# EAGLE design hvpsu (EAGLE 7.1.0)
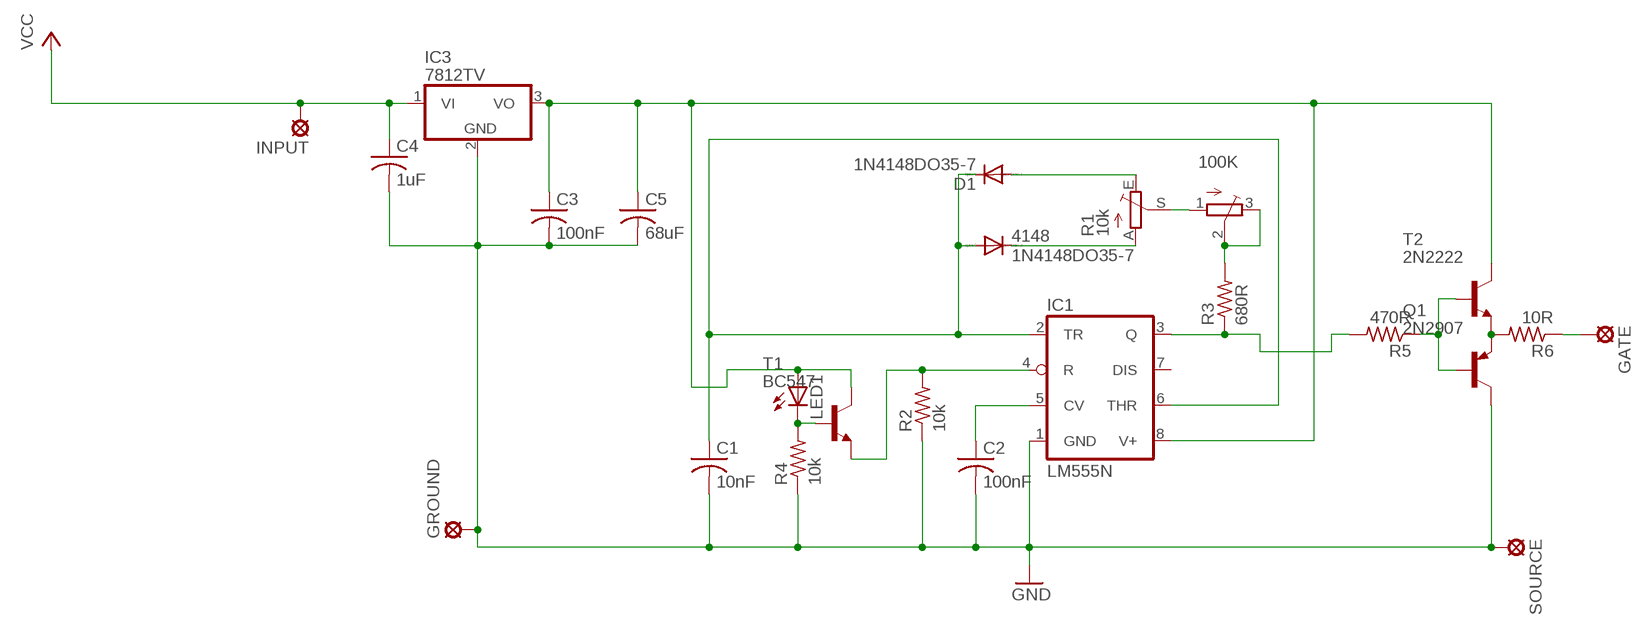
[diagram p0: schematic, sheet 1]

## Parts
100K  TRIMPOT3386  [TRIM-3386]
4148  1N4148DO35-7  [DO35-7]
C1  10nF  C-US050-024X044  [C050-024X044]
C2  100nF  C-US050-024X044  [C050-024X044]
C3  100nF  C-US025-025X050  [C025-025X050]
C4  1uF  C-US025-025X050  [C025-025X050]
C5  68uF  C-US025-025X050  [C025-025X050]
D1  1N4148DO35-7  [DO35-7]
GATE  LSP10  [LSP10]
GROUND  LSP10  [LSP10]
IC1  LM555N  [DIL08-ROUND]
IC3  7812TV  [TO220V]
INPUT  LSP10  [LSP10]
LED1  LED5MM  [LED5MM]
Q1  2N2907  [TO92-EBC-OVAL]
R1  10k  TRIM_EU-S64W  [S64W]
R2  10k  R-US_0204/7  [0204/7]
R3  680R  R-US_0204/7  [0204/7]
R4  10k  R-US_0204/7  [0204/7]
R5  470R  R-US_0204/7  [0204/7]
R6  10R  R-US_0204/7  [0204/7]
SOURCE  LSP10  [LSP10]
T1  BC547  [TO92]
T2  2N2222  [TO92-EBC-OVAL]

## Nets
4148: 4148.A C1.1 D1.C IC1.2(TR) IC1.6(THR)
GND: C1.2 C2.2 C3.2 C4.2 C5.2 GROUND.MP IC1.1(GND) IC3.2(GND) Q1.C R2.1 R4.1 SOURCE.MP
N$1: C2.1 IC1.5(CV)
N$2: IC1.3(Q) R3.1 R5.2
N$3: 100K.2(S) 100K.3(E) R3.2
N$4: 100K.1(A) R1.S
N$5: C3.1 C5.1 IC1.8(V+) IC3.3(VO) LED1.A T1.3(C) T2.C
N$6: 4148.C R1.A
N$7: D1.A R1.E
N$8: LED1.K(C) R4.2 T1.2(B)
N$9: IC1.4(R) R2.2 T1.1(E)
N$10: Q1.B R5.1 T2.B
N$11: Q1.E R6.2 T2.E
N$12: GATE.MP R6.1
VCC: C4.1 IC3.1(VI) INPUT.MP
Unconnected: IC1.7(DIS)

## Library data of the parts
100K = adafruit:TRIMPOT: SMT trimmer potentiometer part number TC33X http://www.ladyada.net/library/eagle
4148 D1 = diode:1N4148: DIODE
C1-C5 = adafruit:C-US: CAPACITOR, American symbol
GATE GROUND INPUT SOURCE = solpad:LSP10: SOLDER PAD
IC1 = adafruit:*555: TIMER Changed DIP package to have round (not oval) pin pads http://www.ladyada.net/library/pcb/eaglelibrary.html
IC3 = linear:78*: Positive VOLTAGE REGULATOR Source: http://cache.national.com/ds/LM/LM78L05.pdf http://www.fairchildsemi.com/ds/LM/LM7805.pdf
LED1 = adafruit:LED: LED
Q1 = adafruit:2N2907*: PNP Transistor Big Oval pads
R1 = pot:TRIM_EU-: POTENTIOMETER
R2-R6 = adafruit:R-US_: RESISTOR, American symbol
T1 = transistor:BC547: NPN TRANSISTOR
T2 = adafruit:2N2222: NPN TRANSISTOR Big oval pads

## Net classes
0 default: clearance 0.508 mm

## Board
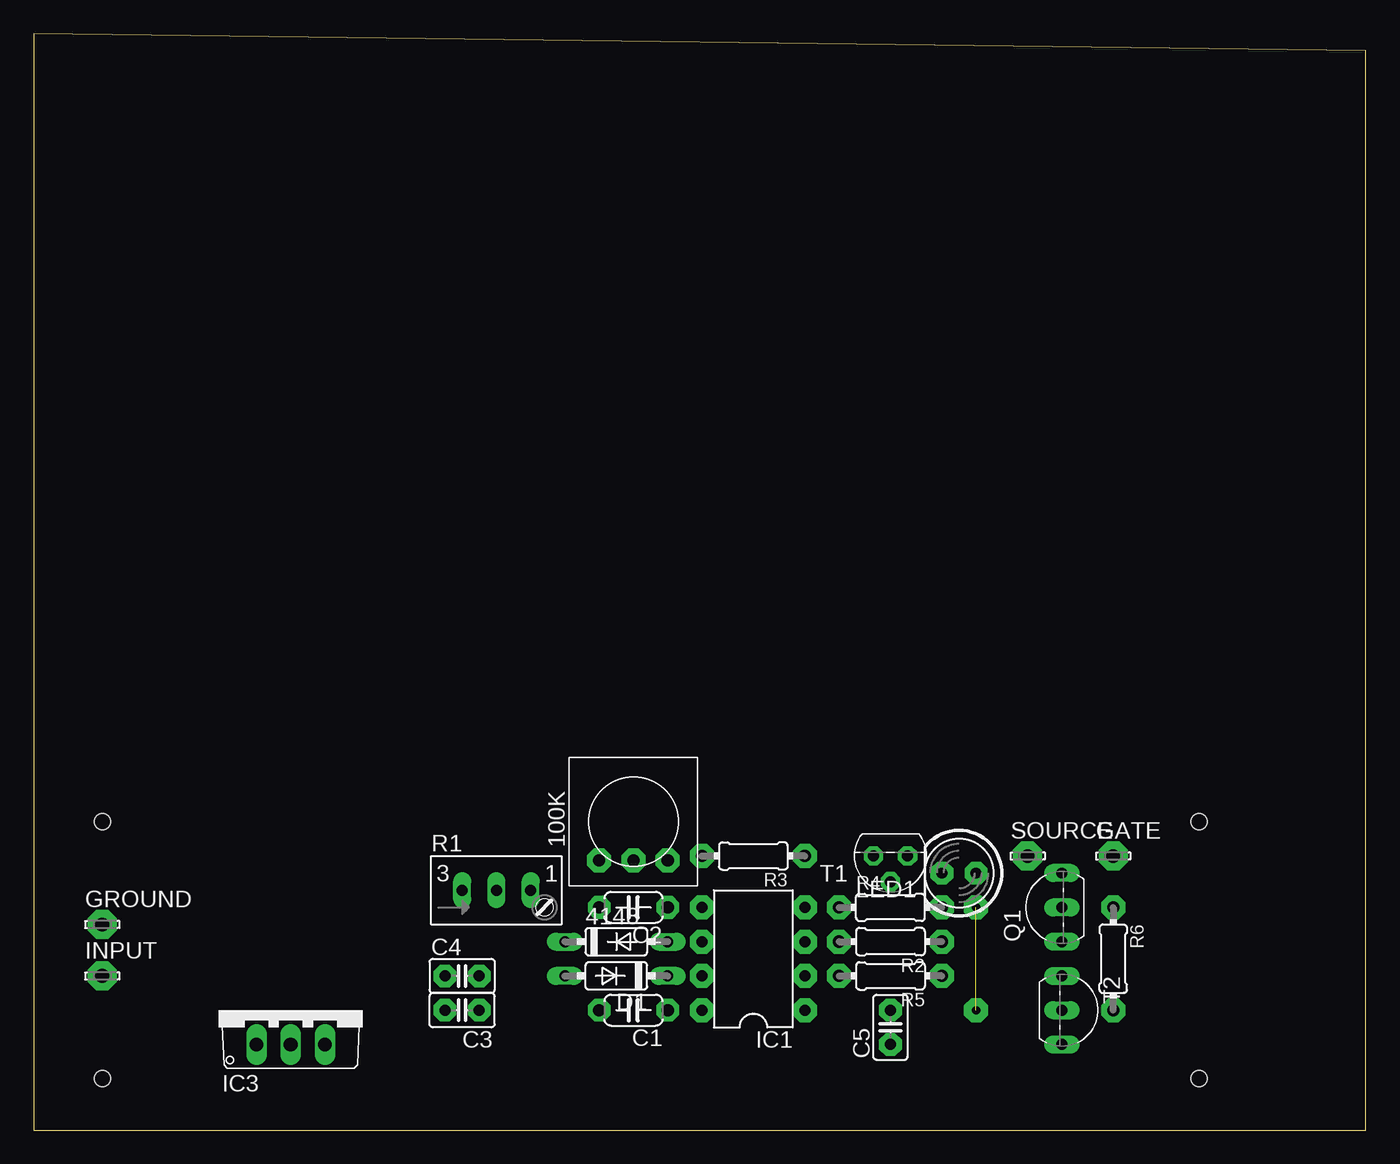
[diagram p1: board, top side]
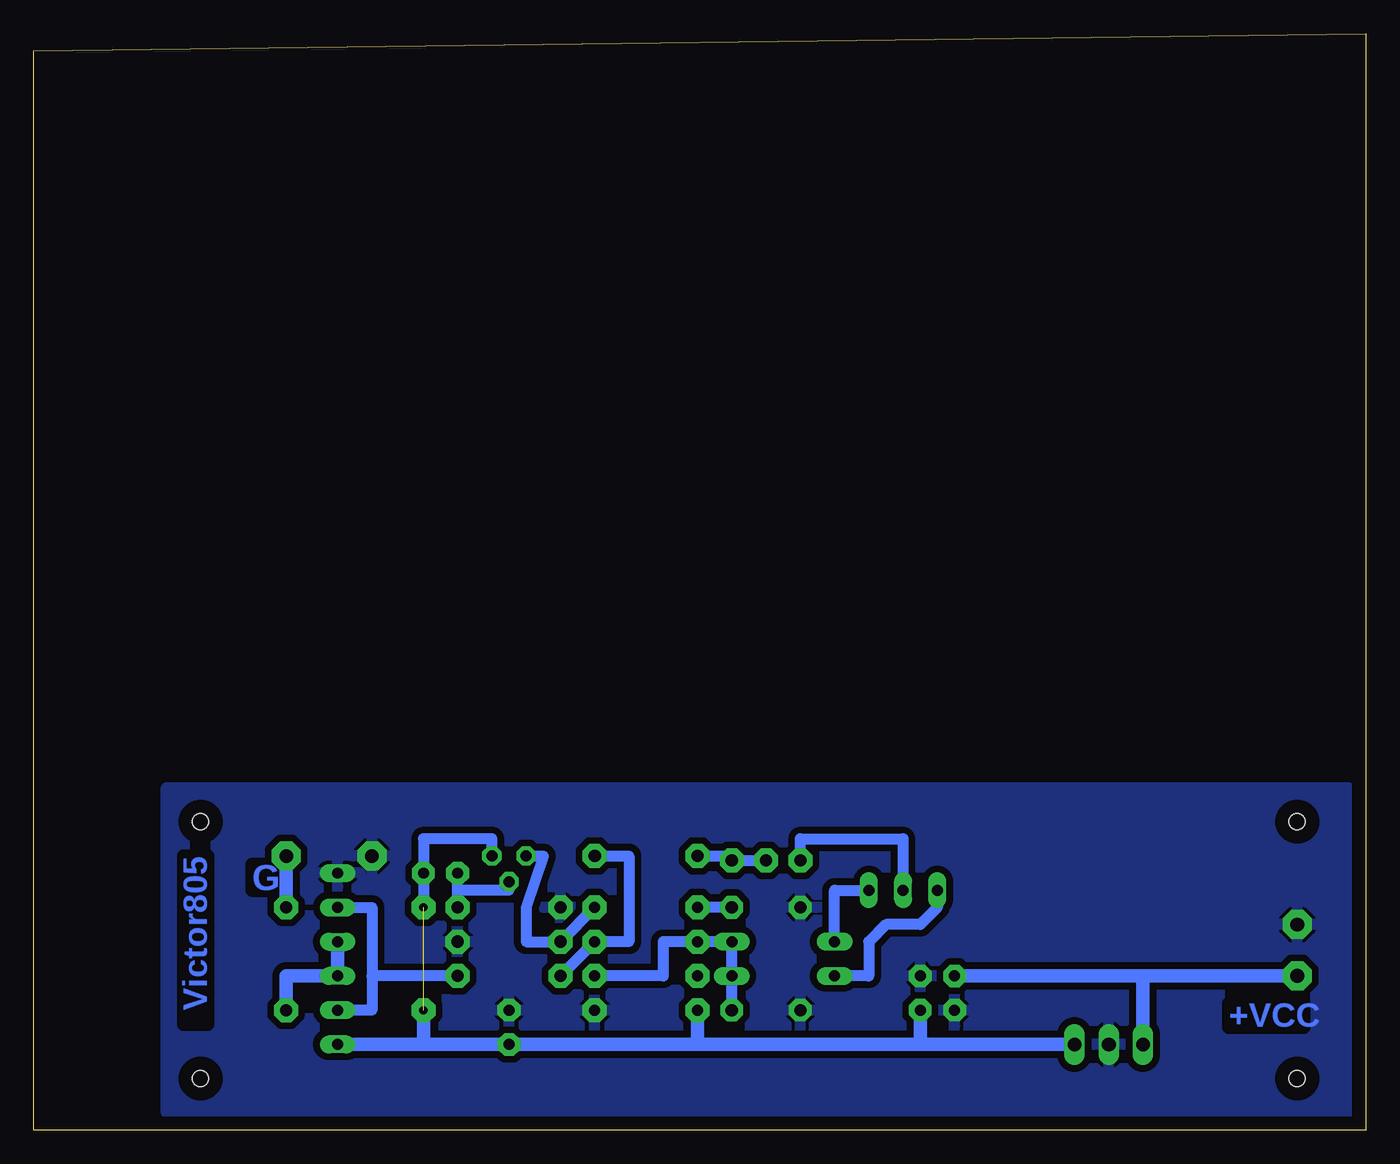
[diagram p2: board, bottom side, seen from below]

Size 98.73 x 81.27 mm. Coordinates in mm from the lower left corner, seen from the top.
Outline: 0,0 98.73,0 98.73,80 0,81.27 0,0
Copper layers (1*16): Top 0.035mm / dielectric 1.5mm / Bottom 0.035mm
Design rules "default": minimum track width 10mil, minimum drill 24mil, track to track 8mil, track to pad 8mil, pad to pad 8mil, via to via 8mil, smd to smd 8mil, copper to edge 40mil, drill to drill 8mil, minimum pad ring 10mil, minimum via ring 8mil, stop-mask expansion 4mil, vias tented up to drill 0mil, thermal gap 10mil
Holes 1.2 mm at 5.08,22.86 5.08,3.81 86.36,22.86 86.36,3.81

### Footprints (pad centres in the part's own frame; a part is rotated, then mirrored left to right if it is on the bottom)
TRIM-3386 = drill 0.9 pad 1.778 octagon: 1 -2.54,-2.857; 2 0,-2.857; 3 2.54,-2.857
DO35-7 = drill 0.813 long: A 3.81,0; C -3.81,0
C050-024X044 = drill 0.9 pad 1.676 octagon: 1 -2.54,0; 2 2.54,0
C025-025X050 = drill 0.813 pad 1.676 octagon: 1 -1.27,0; 2 1.27,0
LSP10 = drill 1.016 pad 2.159 octagon: MP 0,0
DIL08-ROUND = drill 0.813 pad 1.778 octagon: 1 -3.81,-3.81; 2 -1.27,-3.81; 3 1.27,-3.81; 4 3.81,-3.81; 5 3.81,3.81; 6 1.27,3.81; 7 -1.27,3.81; 8 -3.81,3.81
TO220V = drill 1.016 long: 1 -2.54,-2.54; 2 0,-2.54; 3 2.54,-2.54
LED5MM = drill 0.813 pad 1.676 octagon: A -1.27,0; K 1.27,0
TO92-EBC-OVAL = drill 0.813 long: B 0,-1.27; C 2.54,-1.27; E -2.54,-1.27
S64W = drill 0.813 long: A 2.54,1.27; E -2.54,1.27; S 0,1.27
0204/7 = drill 0.9 pad 1.778 octagon: 1 -3.81,0; 2 3.81,0
TO92 = drill 0.813 pad 1.422 octagon: 1 1.27,0; 2 0,1.905; 3 -1.27,0

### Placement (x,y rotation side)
100K  44.45,22.86 0 top
4148  43.18,13.97 0 top
C1  44.45,8.89 180 top
C2  44.45,16.51 180 top
C3  31.75,8.89 180 top
C4  31.75,11.43 0 top
C5  63.5,7.62 90 top
D1  43.18,11.43 180 top
GATE  80.01,20.32 0 top
GROUND  5.08,15.24 0 top
IC1  53.34,12.7 90 top
IC3  19.05,8.89 0 top
INPUT  5.08,11.43 0 top
LED1  68.58,19.05 180 top
Q1  74.93,16.51 90 top
R1  34.29,16.51 0 top
R2  63.5,13.97 180 top
R3  53.34,20.32 180 top
R4  63.5,16.51 0 top
R5  63.5,11.43 180 top
R6  80.01,12.7 270 top
SOURCE  73.66,20.32 0 top
T1  63.5,20.32 180 top
T2  77.47,8.89 270 top

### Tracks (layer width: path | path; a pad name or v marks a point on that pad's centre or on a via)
4148
  Bottom 0.813: IC1.2 52.07,11.43 52.07,13.97 IC1.6 4148.A D1.C C1.1
GND
  pour Bottom: 1.27,25.4 1.27,1.27 88.9,1.27 88.9,25.4
N$1
  Bottom 0.813: C2.1 IC1.5
N$2
  Bottom 0.813: R3.1 54.61,20.32 54.61,13.97 IC1.3 R5.2
N$3
  Bottom 0.813: R3.2 46.99,20.32 100K.3 100K.2
N$4
  Bottom 0.813: 41.91,20.32 100K.1 41.91,21.59 34.29,21.59 R1.S
N$5  (via drill 0.6 pad 1.78)  (1 unrouted)
  Bottom 0.813: v69.85,16.51 LED1.A 69.85,21.59 64.77,21.59 T1.3
  Bottom 1.016: IC1.8 49.53,6.35 | 49.53,6.35 C5.1 69.85,6.35 | 69.85,6.35 T2.C | C3.1 33.02,6.35 | 33.02,6.35 49.53,6.35 | v69.85,8.89 69.85,6.35 | IC3.3 33.02,6.35
N$6
  Bottom 0.813: 4148.C 39.37,17.78 R1.A
N$7
  Bottom 0.813: R1.E 31.75,16.51 33.02,15.24 35.56,15.24 36.83,13.97 36.83,11.43 D1.A
N$8
  Bottom 0.813: R4.2 67.31,17.78 | 67.31,17.78 LED1.K | T1.2 63.5,17.78 67.31,17.78
N$9
  Bottom 0.813: IC1.4 R2.2 62.23,13.97 62.23,16.51 60.96,20.32 T1.1
N$10
  Bottom 0.813: Q1.B 73.66,16.51 73.66,11.43 | 73.66,11.43 73.66,8.89 T2.B | R5.1 73.66,11.43
N$11
  Bottom 1.016: Q1.E T2.E 80.01,11.43 R6.2
N$12
  Bottom 1.016: R6.1 GATE.MP
VCC
  Bottom 1.016: IC3.1 16.51,11.43 | 16.51,11.43 C4.1 | INPUT.MP 16.51,11.43

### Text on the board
Bottom: Victor805 | G | +VCC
